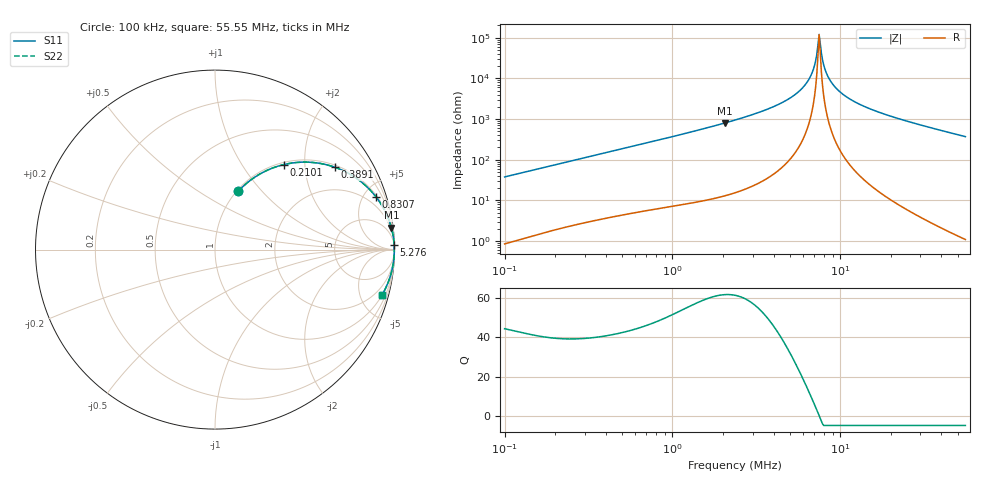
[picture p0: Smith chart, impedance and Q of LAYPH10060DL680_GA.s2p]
! LAYPH10060DL680_GA  S-PARAMETER MODEL  ( General Type )
! Model Generated by TAIYO YUDEN Corporation (http://www.ty-top.com)
! Version 3.0
! TAIYO YUDEN Control No. 180828NI43SB-FBB
! Copyright(c) 2017 TAIYO YUDEN CO.,LTD. All Rights Reserved.
! Product Description (link to TY-COMPAS)
! https://ds.yuden.co.jp/TYCOMPAS/or/detail?pn=LAYPH10060DL680MGA&u=M
! Products Name : Inductors
! Characteristics :
!  Inductance : 68 uH , SRF(min) : -Hz , DC Resistance(max) : 0.121 Ohm
!  Rated Current : Saturation :1.7 A , Temp Rise : 1.3 A (25 degC)
!  Case Size : 10.1 x 10.0 / 0.398 x 0.394 [mm/inch] , Thickness : 6 / 0.236 [mm/inch]
!  (Conditions: Temperature = 25 degC , DC Bias Current/Voltage = 0A / 0V)
! External Node Assignments :
!  1  o---GGG---o  2
! GND o---------o GND
! Frequency Range : 0.1MHz  -  55.545741MHz  [ 402 STEP ]
# MHz S RI R 50
! Freq[MHz].  S11 Real  S11 Imag  S21 Real  S21 Imag  S12 Real  S12 Imag  S22 Real  S22 Imag
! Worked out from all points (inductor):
!   401 points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, 100 kHz to 55.55 MHz, reference 50 ohm
!   read as one part in series: L = 59.7 uH near 103.2 kHz
!   highest Q = 61.9 at 2.044 MHz (marker M1), where L = 62 uH
!   self-resonance near 7.468 MHz
!   S11 on the Smith chart (normalised r, x): 100 kHz: 1.02, +0.75; 210.1 kHz: 1.04, +1.56; 389.1 kHz: 1.07, +2.87; 830.7 kHz: 1.13, +6.11; 5.276 MHz: 4, +75; 55.55 MHz: 1.02, -7.37
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0.1  0.1297 0.3249  0.8703 -0.3249  0.8703 -0.3249  0.1297 0.3249
0.210134  0.3826 0.4735  0.6174 -0.4735  0.6174 -0.4735  0.3826 0.4735
0.288223  0.5317 0.4865  0.4683 -0.4865  0.4683 -0.4865  0.5317 0.4865
0.389135  0.6691 0.4584  0.3309 -0.4584  0.3309 -0.4584  0.6691 0.4584
0.830726  0.8984 0.292  0.1016 -0.292  0.1016 -0.292  0.8984 0.292
2.044423  0.9825 0.1231  0.0175 -0.1231  0.0175 -0.1231  0.9825 0.1231
2.394347  0.9877 0.1026  0.0123 -0.1026  0.0123 -0.1026  0.9877 0.1026
3.846235  0.9961 0.0529  0.00392 -0.0529  0.00392 -0.0529  0.9961 0.0529
5.275557  0.9984 0.0264  0.00163 -0.0264  0.00163 -0.0264  0.9984 0.0264
6.178522  0.9989 0.0142  0.00108 -0.0142  0.00108 -0.0142  0.9989 0.0142
6.792887  0.9991 0.00714  0.0009 -0.00714  0.0009 -0.00714  0.9991 0.00714
7.010962  0.9991 0.00478  0.000864 -0.00478  0.000864 -0.00478  0.9991 0.00478
7.351272  0.9992 0.00126  0.000832 -0.00126  0.000832 -0.00126  0.9992 0.00126
7.468341  0.9992 8.84e-05  0.000827 -8.84e-05  0.000827 -8.84e-05  0.9992 8.84e-05
7.708101  0.9992 -0.00226  0.000826 0.00226  0.000826 0.00226  0.9992 -0.00226
7.955558  0.9992 -0.00461  0.000836 0.00461  0.000836 0.00461  0.9992 -0.00461
8.341719  0.9991 -0.00814  0.000873 0.00814  0.000873 0.00814  0.9991 -0.00814
8.885913  0.999 -0.0129  0.000963 0.0129  0.000963 0.0129  0.999 -0.0129
9.616348  0.9989 -0.0189  0.00114 0.0189  0.00114 0.0189  0.9989 -0.0189
12.57934  0.9976 -0.0403  0.00239 0.0403  0.00239 0.0403  0.9976 -0.0403
19.57868  0.9924 -0.0825  0.0076 0.0825  0.0076 0.0825  0.9924 -0.0825
55.54574  0.9308 -0.2523  0.0692 0.2523  0.0692 0.2523  0.9308 -0.2523
